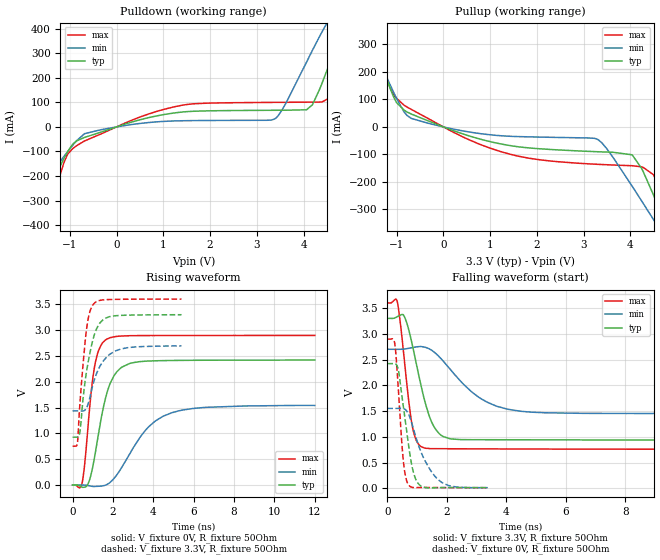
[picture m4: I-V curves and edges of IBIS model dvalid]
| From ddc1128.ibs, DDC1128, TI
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|   dvalid Model
[Model]   dvalid
Model_type   Output
Polarity   Non-Inverting
Vmeas = 1.65
Vref = 0
Cref = 5pF
Rref = 100
|   typ   min   max
|   (nom PVT)   (fast PVT)   (slow PVT)
C_comp   7.826e-12   7.251e-12   8.375e-12
| Where nom  PVT is Nominal Process, 3.3V, 27C
|   Fast PVT is Strong Process,  3.6V, -40C
|   Slow PVT is Weak Process,   2.7V, 125C
[Voltage Range]   3.3   2.7   3.6
|Junction Temperature
[Temperature Range]   27   125   -40
[Pullup Reference]   3.3   2.7   3.6
[Pulldown Reference]   0   0   0
[Power Clamp Reference]   3.3   2.7   3.6
[GND Clamp Reference]   0   0   0
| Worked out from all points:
|   slope of the pulldown table from 0 to 0.495 V, typ, clamps not added: 17.2 ohm
|   slope of the pullup table from 0 to 0.495 V, typ, clamps not added: 16.7 ohm
|   falling waveform, V_fixture 3.3V, R_fixture 50Ohm: 20-80 % time 585ps typ, 1.37ns min, 333ps max; typ from 3.3 V to 0.93 V
|   rising waveform, V_fixture 0V, R_fixture 50Ohm: 20-80 % time 766ps typ, 1.7ns min, 459ps max; typ from 0 V to 2.42 V
|   rising waveform, V_fixture 3.3V, R_fixture 50Ohm: 20-80 % time 558ps typ, 755ps min, 376ps max; typ from 0.926 V to 3.3 V
|   falling waveform, V_fixture 0V, R_fixture 50Ohm: 20-80 % time 350ps typ, 653ps min, 205ps max; typ from 2.42 V to 0.012 V
[Pulldown]
|   Voltage   I(typ)   I(min)   I(max)
-3.3V     -1.023A    -698.6mA   -1.559A
-1.67V    -344.3mA   -261.4mA   -481.9mA
-1.059V   -105.4mA   -103.8mA   -116.1mA
-683.7mV  -42.63mA   -27.46mA   -57.03mA
1.252V    57.47mA    24.52mA    82.71mA
3.385V    67.95mA    32.74mA    100.2mA
4.066V    69.95mA    264.4mA    101mA
4.192V    90.94mA    313mA      101.1mA
4.544V    251.9mA    438.2mA    117mA
4.796V    376.2mA    516.1mA    256.9mA
5.013V    474.8mA    574.8mA    394.4mA
6.6V      887.7mA    844.3mA    957.4mA
[Pullup]
|   Voltage   I(typ)   I(min)   I(max)
-3.3V     814.6mA    736.3mA    895.7mA
-1.729V   414.5mA    373mA      473.4mA
-1.09V    119.1mA    134.7mA    123.3mA
-686.4mV  46.85mA    31mA       63.7mA
1.251V    -62.62mA   -32.34mA   -90.98mA
3.312V    -90.3mA    -46.59mA   -136.1mA
4.039V    -101.5mA   -215.8mA   -141.1mA
4.494V    -247.3mA   -336.9mA   -173.8mA
4.602V    -290.9mA   -365.9mA   -212.4mA
4.778V    -363.2mA   -413.4mA   -313.7mA
4.864V    -398.7mA   -436.6mA   -367.4mA
6.6V      -1.127A    -906.3mA   -1.512A
[Ramp]
R_load = 50
|   typ   min   max
dV/dt_r   1.45187/7.67354e-10   0.926941/1.70336e-09   1.73782/4.59257e-10
dV/dt_f   1.42179/5.85201e-10   0.75383/1.36673e-09   1.70797/3.3243e-10
[Falling Waveform]
V_fixture = 3.3V
V_fixture_min = 2.7V
V_fixture_max = 3.6V
R_fixture = 50Ohm
|   Time   V(typ)   V(min)   V(max)
0s        3.3V       2.7V       3.6V
325ps     3.33V      2.7V       3.645V
550ps     3.36V      2.704V     2.61V
825ps     2.823V     2.731V     1.253V
975ps     2.417V     2.746V     925.2mV
1.25ns    1.712V     2.741V     781.6mV
1.875ns   1.005V     2.472V     768mV
3.125ns   943mV      1.747V     764.8mV
4.475ns   941.5mV    1.496V     762.4mV
20ns      930.3mV    1.444V     753.4mV
[Rising Waveform]
V_fixture = 0V
V_fixture_min = 0V
V_fixture_max = 0V
R_fixture = 50Ohm
|   Time   V(typ)   V(min)   V(max)
0s        3.066nV    4.992nV    2.613nV
475ps     -42.34mV   494.1uV    41.84mV
800ps     52.24mV    -12.18mV   1.292V
975ps     303.8mV    -25.29mV   1.977V
1.15ns    672.3mV    -26.42mV   2.406V
1.65ns    1.708V     1.019mV    2.812V
2.45ns    2.283V     349.3mV    2.884V
3.65ns    2.397V     1.076V     2.893V
4.9ns     2.41V      1.397V     2.893V
12ns      2.418V     1.541V     2.895V
[Rising Waveform]
V_fixture = 3.3V
V_fixture_min = 2.7V
V_fixture_max = 3.6V
R_fixture = 50Ohm
|   Time   V(typ)   V(min)   V(max)
0s        926.4mV    1.435V     752mV
250ps     927.5mV    1.435V     843.9mV
375ps     1.056V     1.434V     1.635V
525ps     1.687V     1.433V     2.354V
650ps     2.086V     1.465V     2.871V
800ps     2.433V     1.606V     3.264V
1ns       2.798V     1.926V     3.481V
1.375ns   3.146V     2.312V     3.575V
2.125ns   3.276V     2.595V     3.593V
5.4ns     3.296V     2.692V     3.598V
[Falling Waveform]
V_fixture = 0V
V_fixture_min = 0V
V_fixture_max = 0V
R_fixture = 50Ohm
|   Time   V(typ)   V(min)   V(max)
0s        2.422V     1.551V     2.897V
250ps     2.423V     1.551V     2.814V
375ps     2.28V      1.552V     1.88V
525ps     1.644V     1.55V      608.7mV
600ps     1.327V     1.531V     265.4mV
700ps     895.8mV    1.455V     77.49mV
850ps     371.3mV    1.212V     14.61mV
1ns       122.1mV    916.7mV    12.46mV
1.725ns   11.5mV     158.4mV    12.82mV
3.375ns   12.02mV    11.13mV    10.11mV
